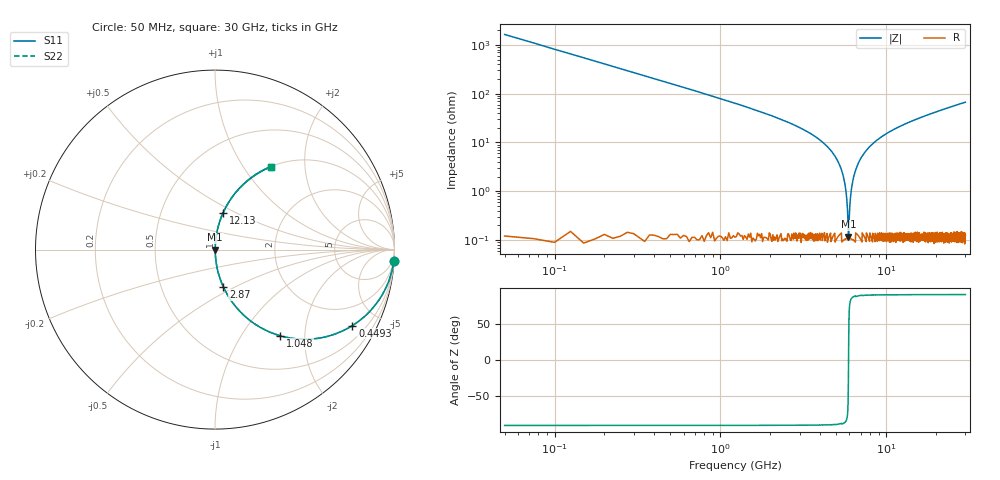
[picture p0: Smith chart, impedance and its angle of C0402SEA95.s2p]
!	AVX Thin Film Operation 	Date: April 2014
!	Description: Accu-P® Series, Thin Film  SMD RF Capacitor
!	Part Number: 04021JA95ZBSTR
# MHZ S MA R 50
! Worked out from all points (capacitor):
!   1201 points, 50 MHz to 30 GHz, reference 50 ohm
!   read as one part in series: C = 1.95 pF near 199.8 MHz
!   lowest |Z| = 117 mohm at 5.915 GHz (marker M1)
!   series resonance near 5.925 GHz, so ESL is about 370 pH
!   S11 on the Smith chart (normalised r, x): 50 MHz: 1, -33; 449.3 MHz: 1.00, -3.61; 1.048 GHz: 1.00, -1.51; 2.87 GHz: 1.00, -0.43; 12.13 GHz: 1.00, +0.43; 30 GHz: 1.00, +1.34
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50  0.998 -3.5  0.061 86.5  0.061 86.5  0.998 -3.5
274.625  0.947 -18.6  0.319 71.3  0.319 71.3  0.947 -18.6
449.333  0.875 -29.0  0.484 61.0  0.484 61.0  0.875 -29.0
1048.333  0.602 -52.9  0.798 37.0  0.798 37.0  0.602 -52.9
1772.125  0.386 -67.1  0.921 22.7  0.921 22.7  0.386 -67.1
2870.292  0.212 -77.4  0.976 12.3  0.976 12.3  0.212 -77.4
5041.667  0.045 -86.0  0.998 2.6  0.998 2.6  0.045 -86.0
5540.833  0.018 -85.3  0.999 1.1  0.999 1.1  0.018 -85.3
5690.583  0.011 -83.4  0.999 0.6  0.999 0.6  0.011 -83.4
5815.375  0.005268 -77.0  0.999 0.3  0.999 0.3  0.005268 -77.0
5915.208  0.001245 -21.4  0.999 0.0  0.999 0.0  0.001245 -21.4
6015.042  0.00431 74.2  0.999 -0.2  0.999 -0.2  0.00431 74.2
6164.792  0.011 83.3  0.999 -0.6  0.999 -0.6  0.011 83.3
6339.5  0.019 85.4  0.999 -1.1  0.999 -1.1  0.019 85.4
6938.5  0.044 86.0  0.998 -2.5  0.998 -2.5  0.044 86.0
8161.458  0.089 84.1  0.995 -5.1  0.995 -5.1  0.089 84.1
10058.29  0.151 80.9  0.987 -8.7  0.987 -8.7  0.151 80.9
12129.83  0.21 77.6  0.977 -12.1  0.977 -12.1  0.21 77.6
15025  0.283 73.4  0.958 -16.4  0.958 -16.4  0.283 73.4
20016.67  0.39 66.9  0.92 -23.0  0.92 -23.0  0.39 66.9
25033.29  0.481 61.1  0.876 -28.8  0.876 -28.8  0.481 61.1
30000  0.556 56.1  0.83 -33.8  0.83 -33.8  0.556 56.1
